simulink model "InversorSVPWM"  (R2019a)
settings: Solver=ode23t  StartTime=0.0  StopTime=0.06  RelTol=1e-3
libraries: powerlib x22, powerlib_meascontrol x6, simulink x3

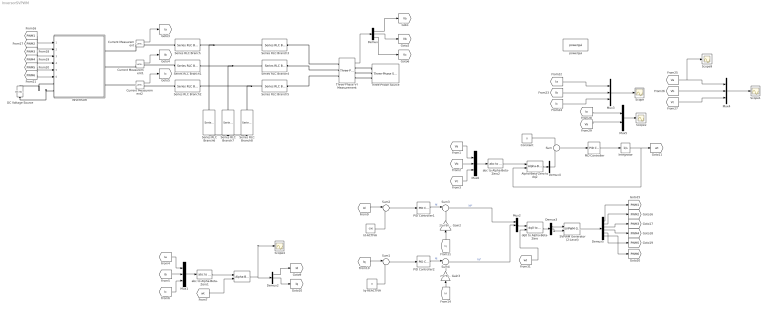
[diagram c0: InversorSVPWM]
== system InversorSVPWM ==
  " " : powerlib_meascontrol/Transformations/Alpha-Beta-Zero to dq0  Alignment=90 degrees behind phase A axis
  Alpha-Beta-Zero to dq2 : powerlib_meascontrol/Transformations/Alpha-Beta-Zero to dq0  Alignment=90 degrees behind phase A axis
  Constant : Constant  Value=0
  Current Measurement : powerlib/Measurements/Current Measurement  PhasorSimulation=off  OutputType=Complex  PSBequivalent=0
  Current Measurement1 : powerlib/Measurements/Current Measurement  PhasorSimulation=off  OutputType=Complex  PSBequivalent=0
  Current Measurement2 : powerlib/Measurements/Current Measurement  PhasorSimulation=off  OutputType=Complex  PSBequivalent=0
  DC Voltage Source : powerlib/Electrical Sources/DC Voltage Source  Amplitude=800  Measurements=None
  Demux{,2..4} (4 alike) : Demux  Outputs=3
  Demux5 : Demux  Outputs=6
  Gain2 : Gain  Gain=2*pi*50*1000e-6
  Gain3 : Gain  Gain=2*pi*50*1000e-6
  INVERSOR : Subsystem
  "Id-ACTIVA " : Constant  Value=-100
  Integrator : Integrator
  Iq-REACTIVA : Constant  Value=0
  Mux{1..4,6} (5 alike) : Mux  Inputs=3
  Mux5 : Mux  Inputs=2
  PID Controller : simulink/Continuous/PID Controller  Controller=PI  Form=Parallel  TimeDomain=Continuous-time  SampleTime=-1  IntegratorMethod=Forward Euler  FilterMethod=Forward Euler  ControllerParametersSource=internal  P=10  I=50000  D=0  UseFilter=on  N=100  TunerSelectOption=Transfer Function Based (PID Tuner App)  InitialConditionSource=internal  InitialConditionForIntegrator=0  InitialConditionForFilter=0  DifferentiatorICPrevScaledInput=0  ExternalReset=none  TrackingMode=off  Kt=1  LimitOutput=off  UpperSaturationLimit=inf  LowerSaturationLimit=-inf  LinearizeAsGain=on  AntiWindupMode=none  Kb=1  POutMin=[]  POutMax=[]  IOutMin=[]  IOutMax=[]  DOutMin=[]  DOutMax=[]  NOutMin=[]  NOutMax=[]  SumOutMin=[]  SumOutMax=[]  SaturationOutMin=[]  SaturationOutMax=[]  PParamMin=[]  PParamMax=[]  IParamMin=[]  IParamMax=[]  DParamMin=[]  DParamMax=[]  NParamMin=[]  NParamMax=[]  KbParamMin=[]  KbParamMax=[]  KtParamMin=[]  KtParamMax=[]  KbOutMin=[]  KbOutMax=[]  KtOutMin=[]  KtOutMax=[]  IntegratorOutMin=[]  IntegratorOutMax=[]  FilterOutMin=[]  FilterOutMax=[]  SumI1OutMin=[]  SumI1OutMax=[]  SumI2OutMin=[]  SumI2OutMax=[]  SumI3OutMin=[]  SumI3OutMax=[]  SumI4OutMin=[]  SumI4OutMax=[]  SumDOutMin=[]  SumDOutMax=[]  DifferentiatorOutMin=[]  DifferentiatorOutMax=[]  FilterDiffOutCoefMin=[]  FilterDiffOutCoefMax=[]  ReciprocalOutMin=[]  ReciprocalOutMax=[]  SumDenOutMin=[]  SumDenOutMax=[]  SumNumOutMin=[]  SumNumOutMax=[]  DivideOutMin=[]  DivideOutMax=[]  IntegratorContinuousStateAttributes=''  IntegratorStateMustResolveToSignalObject=off  IntegratorRTWStateStorageClass=Auto  FilterContinuousStateAttributes=''  FilterStateMustResolveToSignalObject=off  FilterRTWStateStorageClass=Auto  ParallelPVariant=InternalParameters  IdealPVariant=Disabled  IVariant=InternalParameters  DVariant=Disabled  IntegratorVariant=Continuous  SatVariant=Disabled  AWVariant=Passthrough  PCopyVariant=Disabled  TRVariant=Disabled  FdbkBlocksVariant=Forward  IdealPFdbkVariant=Disabled  SatFdbkVariant=Disabled  DerivativeFilterVariant=Disabled  NVariant=Disabled  NCopyVariant=Disabled_SignalSpec  FilterICVariant=Disabled  IntegratorICVariant=InternalICs  ExternalResetVariant=Disabled  TRSumVariant=Passthrough  SumFdbkVariant=Disabled  SumVariant=Sum_PI
  PID Controller1 : simulink/Continuous/PID Controller  Controller=PI  Form=Parallel  TimeDomain=Continuous-time  SampleTime=-1  IntegratorMethod=Forward Euler  FilterMethod=Forward Euler  ControllerParametersSource=internal  P=5  I=5000  D=0  UseFilter=on  N=100  TunerSelectOption=Transfer Function Based (PID Tuner App)  InitialConditionSource=internal  InitialConditionForIntegrator=0  InitialConditionForFilter=0  DifferentiatorICPrevScaledInput=0  ExternalReset=none  TrackingMode=off  Kt=1  LimitOutput=off  UpperSaturationLimit=inf  LowerSaturationLimit=-inf  LinearizeAsGain=on  AntiWindupMode=none  Kb=1  POutMin=[]  POutMax=[]  IOutMin=[]  IOutMax=[]  DOutMin=[]  DOutMax=[]  NOutMin=[]  NOutMax=[]  SumOutMin=[]  SumOutMax=[]  SaturationOutMin=[]  SaturationOutMax=[]  PParamMin=[]  PParamMax=[]  IParamMin=[]  IParamMax=[]  DParamMin=[]  DParamMax=[]  NParamMin=[]  NParamMax=[]  KbParamMin=[]  KbParamMax=[]  KtParamMin=[]  KtParamMax=[]  KbOutMin=[]  KbOutMax=[]  KtOutMin=[]  KtOutMax=[]  IntegratorOutMin=[]  IntegratorOutMax=[]  FilterOutMin=[]  FilterOutMax=[]  SumI1OutMin=[]  SumI1OutMax=[]  SumI2OutMin=[]  SumI2OutMax=[]  SumI3OutMin=[]  SumI3OutMax=[]  SumI4OutMin=[]  SumI4OutMax=[]  SumDOutMin=[]  SumDOutMax=[]  DifferentiatorOutMin=[]  DifferentiatorOutMax=[]  FilterDiffOutCoefMin=[]  FilterDiffOutCoefMax=[]  ReciprocalOutMin=[]  ReciprocalOutMax=[]  SumDenOutMin=[]  SumDenOutMax=[]  SumNumOutMin=[]  SumNumOutMax=[]  DivideOutMin=[]  DivideOutMax=[]  IntegratorContinuousStateAttributes=''  IntegratorStateMustResolveToSignalObject=off  IntegratorRTWStateStorageClass=Auto  FilterContinuousStateAttributes=''  FilterStateMustResolveToSignalObject=off  FilterRTWStateStorageClass=Auto  ParallelPVariant=InternalParameters  IdealPVariant=Disabled  IVariant=InternalParameters  DVariant=Disabled  IntegratorVariant=Continuous  SatVariant=Disabled  AWVariant=Passthrough  PCopyVariant=Disabled  TRVariant=Disabled  FdbkBlocksVariant=Forward  IdealPFdbkVariant=Disabled  SatFdbkVariant=Disabled  DerivativeFilterVariant=Disabled  NVariant=Disabled  NCopyVariant=Disabled_SignalSpec  FilterICVariant=Disabled  IntegratorICVariant=InternalICs  ExternalResetVariant=Disabled  TRSumVariant=Passthrough  SumFdbkVariant=Disabled  SumVariant=Sum_PI
  PID Controller2 : simulink/Continuous/PID Controller  Controller=PI  Form=Parallel  TimeDomain=Continuous-time  SampleTime=-1  IntegratorMethod=Forward Euler  FilterMethod=Forward Euler  ControllerParametersSource=internal  P=5  I=5000  D=0  UseFilter=on  N=100  TunerSelectOption=Transfer Function Based (PID Tuner App)  InitialConditionSource=internal  InitialConditionForIntegrator=0  InitialConditionForFilter=0  DifferentiatorICPrevScaledInput=0  ExternalReset=none  TrackingMode=off  Kt=1  LimitOutput=off  UpperSaturationLimit=inf  LowerSaturationLimit=-inf  LinearizeAsGain=on  AntiWindupMode=none  Kb=1  POutMin=[]  POutMax=[]  IOutMin=[]  IOutMax=[]  DOutMin=[]  DOutMax=[]  NOutMin=[]  NOutMax=[]  SumOutMin=[]  SumOutMax=[]  SaturationOutMin=[]  SaturationOutMax=[]  PParamMin=[]  PParamMax=[]  IParamMin=[]  IParamMax=[]  DParamMin=[]  DParamMax=[]  NParamMin=[]  NParamMax=[]  KbParamMin=[]  KbParamMax=[]  KtParamMin=[]  KtParamMax=[]  KbOutMin=[]  KbOutMax=[]  KtOutMin=[]  KtOutMax=[]  IntegratorOutMin=[]  IntegratorOutMax=[]  FilterOutMin=[]  FilterOutMax=[]  SumI1OutMin=[]  SumI1OutMax=[]  SumI2OutMin=[]  SumI2OutMax=[]  SumI3OutMin=[]  SumI3OutMax=[]  SumI4OutMin=[]  SumI4OutMax=[]  SumDOutMin=[]  SumDOutMax=[]  DifferentiatorOutMin=[]  DifferentiatorOutMax=[]  FilterDiffOutCoefMin=[]  FilterDiffOutCoefMax=[]  ReciprocalOutMin=[]  ReciprocalOutMax=[]  SumDenOutMin=[]  SumDenOutMax=[]  SumNumOutMin=[]  SumNumOutMax=[]  DivideOutMin=[]  DivideOutMax=[]  IntegratorContinuousStateAttributes=''  IntegratorStateMustResolveToSignalObject=off  IntegratorRTWStateStorageClass=Auto  FilterContinuousStateAttributes=''  FilterStateMustResolveToSignalObject=off  FilterRTWStateStorageClass=Auto  ParallelPVariant=InternalParameters  IdealPVariant=Disabled  IVariant=InternalParameters  DVariant=Disabled  IntegratorVariant=Continuous  SatVariant=Disabled  AWVariant=Passthrough  PCopyVariant=Disabled  TRVariant=Disabled  FdbkBlocksVariant=Forward  IdealPFdbkVariant=Disabled  SatFdbkVariant=Disabled  DerivativeFilterVariant=Disabled  NVariant=Disabled  NCopyVariant=Disabled_SignalSpec  FilterICVariant=Disabled  IntegratorICVariant=InternalICs  ExternalResetVariant=Disabled  TRSumVariant=Passthrough  SumFdbkVariant=Disabled  SumVariant=Sum_PI
  SVPWM Generator (2-Level) : powerlib_meascontrol/Pulse & Signal Generators/SVPWM Generator (2-Level)  InputType=alpha-beta components  SwitchingPattern=Pattern #1  Fc=2000  ParUref=[0.8 -30 50]  Ts=0
  Scope{,1..2,4,9} (5 alike) : Scope
  Series RLC Branch{,1..5} (6 alike) : powerlib/Elements/Series RLC Branch  LConnTagsString=__new0  RConnTagsString=__new0  BranchType=L  Resistance=1  Inductance=500e-6  SetiL0=off  InitialCurrent=0  Capacitance=1e-6  Setx0=off  InitialVoltage=0  Measurements=None
  Series RLC Branch6 : powerlib/Elements/Series RLC Branch  LConnTagsString=__new0  RConnTagsString=__new0  BranchType=C  Resistance=1  Inductance=500e-6  SetiL0=off  InitialCurrent=0  Capacitance=100e-9  Setx0=off  InitialVoltage=0  Measurements=None
  Series RLC Branch7 : powerlib/Elements/Series RLC Branch  LConnTagsString=__new0  RConnTagsString=__new0  BranchType=C  Resistance=1  Inductance=500e-6  SetiL0=off  InitialCurrent=0  Capacitance=100e-9  Setx0=off  InitialVoltage=0  Measurements=None
  Series RLC Branch8 : powerlib/Elements/Series RLC Branch  LConnTagsString=__new0  RConnTagsString=__new0  BranchType=C  Resistance=1  Inductance=500e-6  SetiL0=off  InitialCurrent=0  Capacitance=100e-9  Setx0=off  InitialVoltage=0  Measurements=None
  Sum : Sum  Inputs=+-
  Sum1 : Sum  Inputs=|-+
  Sum2 : Sum  Inputs=|-+
  Sum3 : Sum  Inputs=|++
  Sum4 : Sum  Inputs=|+-
  Three-Phase V-I Measurement : powerlib/Measurements/Three-Phase V-I Measurement  VoltageMeasurement=phase-to-phase  SetLabelV=off  LabelV=Vabc  Vpu=off  VpuLL=off  CurrentMeasurement=no  SetLabelI=off  LabelI=Iabc  Ipu=off  Pbase=100e6  Vbase=500e3  OutputType=Complex  PhasorSimulation=off  PSBequivalent=0
  Three-Phase Source : powerlib/Electrical Sources/Three-Phase Source  InternalConnection=Y  VoltagePhases=off  Voltage=415  PhaseAngle=0  Voltage_phases=[25e3 25e3 25e3]/sqrt(3)  PhaseAngles_phases=[0 -120 +120]  Frequency=50  NonIdealSource=on  SpecifyImpedance=off  Resistance=0.001e-3  Inductance=0.001e-9  ShortCircuitLevel=100e6  BaseVoltage=415  XRratio=7  BusType=swing  Pref=10e3  Qref=0  Prefabc=[10e3, 10e3, 10e3]  Qrefabc=[0, 0, 0]  Qmin=-inf  Qmax=inf
  abc to Alpha-Beta-Zero1 : powerlib_meascontrol/Transformations/abc to Alpha-Beta-Zero
  abc to Alpha-Beta-Zero2 : powerlib_meascontrol/Transformations/abc to Alpha-Beta-Zero
  dq0 to Alpha-Beta-Zero : powerlib_meascontrol/Transformations/dq0 to Alpha-Beta-Zero  Alignment=90 degrees behind phase A axis
  powergui : powerlib/powergui  Priority=1  SimulationMode=Discrete  SampleTime=1e-6  frequency=60  Iterations=50  frequencyindice=50  Pbase=100e6  ErrMax=1e-4  UnitsV=kV  UnitsW=MW  buscounter=0  FunctionMessages=off  echomessages=off  EnableUseOfTLC=off  CurrentSourceSwitches=off  DisableSnubberDevices=off  DisableRonSwitches=off  DisableVfSwitches=off  DisplayEquations=off  AutomaticDiscreteSolvers=off  SolverType=Tustin/Backward Euler (TBE)  Interpol=off  ExternalGateDelay=off  methode=off  Ts=100  x0status=blocks  SPID=on  SwTol=0  HookPort=off  NonlinearTolerance=0  nMaxIteration=15  ContinueOnMaxIteration=off  RestoreLinks=warning  ResistiveCurrentMeasurement=off  Frange=[0:2:500]  Ylog=off  Xlog=on  ShowGrid=off  save=off  variable=ZData  structure=0  ZoomFFT=off  StartTime=0.0  cycles=1  DisplayStyle=1  fundamental=60  FreqAxis=off  MaxFrequency=1000  frequencyindicesteady=1  RmsSteady=1  display=off
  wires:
  [PWM6] -> INVERSOR/6(PWM6)
  [PWM2] -> INVERSOR/2(PWM2)
  [PWM5] -> INVERSOR/5(PWM5)
  [PWM3] -> INVERSOR/3(PWM3)
  [Id] -> Gain3/1
  Current Measurement/1 -> [Ia]
  Sum1/1 -> PID Controller2/1
  PID Controller2/1 -> Sum4/1  "Iq"
  Iq-REACTIVA/1 -> Sum1/2
  [Id] -> Sum2/1
  Integrator/1 -> Alpha-Beta-Zero to dq2/2, [wt]
  PID Controller/1 -> Integrator/1
  " "/1 -> Scope4/1, Demux2/1
  [Ib] -> Mux1/2
  Demux2/1 -> [Id]
  [Ic] -> Mux1/3
  Mux1/1 -> abc to Alpha-Beta-Zero1/1
  Sum2/1 -> PID Controller1/1
  [Ia] -> Mux1/1
  Demux2/2 -> [Iq]
  [wt] -> " "/2
  [Iq] -> Gain2/1
  Current Measurement2/1 -> [Ic]
  Current Measurement1/1 -> [Ib]
  Gain3/1 -> Sum4/2
  PID Controller1/1 -> Sum3/1  "Id"
  abc to Alpha-Beta-Zero2/1 -> Alpha-Beta-Zero to dq2/1
  Constant/1 -> Sum/1
  Sum/1 -> PID Controller/1
  [PWM4] -> INVERSOR/4(PWM4)
  [PWM1] -> INVERSOR/1(PWM1)
  Gain2/1 -> Sum3/2
  "Id-ACTIVA "/1 -> Sum2/2
  [Iq] -> Sum1/1
  [Ic] -> Mux3/3
  [Ib] -> Mux3/2
  Mux3/1 -> Scope/1
  Mux4/1 -> Scope1/1
  [Va] -> Scope9/1, Mux4/1
  [Vb] -> Mux4/2
  [Vc] -> Mux4/3
  Alpha-Beta-Zero to dq2/1 -> Demux4/1
  Demux4/2 -> Sum/2
  [Ia] -> Mux5/1
  [Va] -> Mux5/2
  Mux5/1 -> Scope2/1
  [Ia] -> Mux3/1
  dq0 to Alpha-Beta-Zero/1 -> Demux3/1
  SVPWM Generator (2-Level)/1 -> Demux5/1
  Demux3/2 -> SVPWM Generator (2-Level)/2
  [wt] -> dq0 to Alpha-Beta-Zero/2
  Mux2/1 -> dq0 to Alpha-Beta-Zero/1
  Demux3/1 -> SVPWM Generator (2-Level)/1
  Demux5/1 -> [PWM1]
  Demux5/2 -> [PWM2]
  Demux5/3 -> [PWM3]
  Demux5/4 -> [PWM4]
  Demux5/5 -> [PWM5]
  Demux5/6 -> [PWM6]
  Sum3/1 -> Mux2/1  "Id*"
  Sum4/1 -> Mux2/2  "Iq*"
  abc to Alpha-Beta-Zero1/1 -> " "/1
  Demux/3 -> [Vc]
  Demux/2 -> [Vb]
  Three-Phase V-I Measurement/1 -> Demux/1
  Demux/1 -> [Va]
  [Va] -> Mux6/1
  Mux6/1 -> abc to Alpha-Beta-Zero2/1
  [Vc] -> Mux6/3
  [Vb] -> Mux6/2
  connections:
  Series RLC Branch7/RConn1 -- Series RLC Branch6/RConn1 -- Series RLC Branch8/RConn1
  Series RLC Branch5/LConn1 -- Series RLC Branch8/LConn1 -- Series RLC Branch2/RConn1
  Series RLC Branch4/LConn1 -- Series RLC Branch7/LConn1 -- Series RLC Branch1/RConn1
  Series RLC Branch3/LConn1 -- Series RLC Branch6/LConn1 -- Series RLC Branch/RConn1
  Series RLC Branch/LConn1 -- Current Measurement/RConn1
  Series RLC Branch2/LConn1 -- Current Measurement2/RConn1
  Series RLC Branch1/LConn1 -- Current Measurement1/RConn1
  Current Measurement/LConn1 -- INVERSOR/RConn1
  Current Measurement1/LConn1 -- INVERSOR/RConn2
  DC Voltage Source/LConn1 -- INVERSOR/LConn2
  DC Voltage Source/RConn1 -- INVERSOR/LConn1
  INVERSOR/RConn3 -- Current Measurement2/LConn1
  Series RLC Branch3/RConn1 -- Three-Phase V-I Measurement/LConn1
  Series RLC Branch4/RConn1 -- Three-Phase V-I Measurement/LConn2
  Series RLC Branch5/RConn1 -- Three-Phase V-I Measurement/LConn3
  Three-Phase Source/RConn1 -- Three-Phase V-I Measurement/RConn1
  Three-Phase Source/RConn2 -- Three-Phase V-I Measurement/RConn2
  Three-Phase Source/RConn3 -- Three-Phase V-I Measurement/RConn3

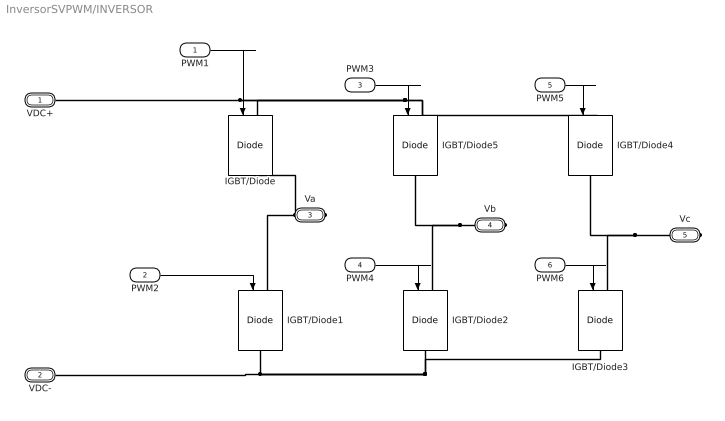
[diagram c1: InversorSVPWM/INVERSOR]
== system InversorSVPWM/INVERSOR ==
  PWM1 : Inport
  PWM2 : Inport  Port=2
  PWM3 : Inport  Port=3
  PWM4 : Inport  Port=4
  PWM5 : Inport  Port=5
  PWM6 : Inport  Port=6
  IGBT/Diode{,1..5} (6 alike) : powerlib/Power Electronics/IGBT//Diode  Ron=1e-3  Rs=1e5  Cs=inf  Measurements=off
  VDC+ : PMIOPort  Side=Left
  VDC- : PMIOPort  Port=2  Side=Left
  Va : PMIOPort  Port=3  Side=Right
  Vb : PMIOPort  Port=4  Side=Right
  Vc : PMIOPort  Port=5  Side=Right
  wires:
  PWM6/1 -> IGBT/Diode3/1
  PWM4/1 -> IGBT/Diode2/1
  PWM5/1 -> IGBT/Diode4/1
  PWM1/1 -> IGBT/Diode/1
  PWM2/1 -> IGBT/Diode1/1
  PWM3/1 -> IGBT/Diode5/1
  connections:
  IGBT/Diode/LConn1 -- VDC+/RConn1 -- IGBT/Diode5/LConn1 -- IGBT/Diode4/LConn1
  IGBT/Diode1/RConn1 -- VDC-/RConn1 -- IGBT/Diode3/RConn1 -- IGBT/Diode2/RConn1
  Vb/RConn1 -- IGBT/Diode5/RConn1 -- IGBT/Diode2/LConn1
  Vc/RConn1 -- IGBT/Diode4/RConn1 -- IGBT/Diode3/LConn1
  Va/RConn1 -- IGBT/Diode1/LConn1 -- IGBT/Diode/RConn1
